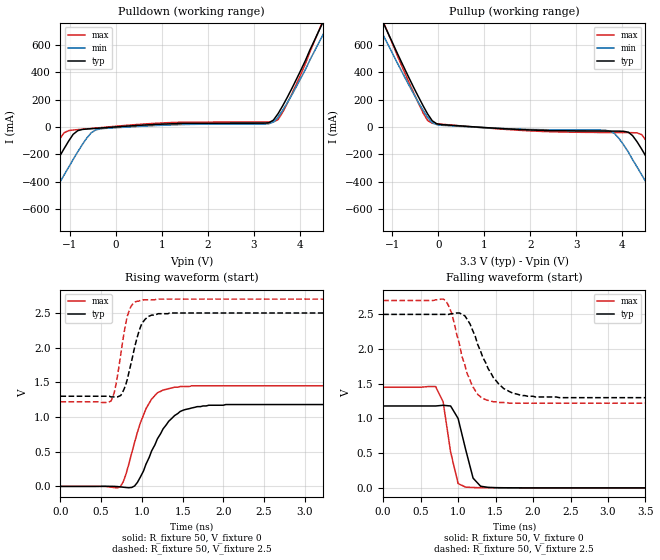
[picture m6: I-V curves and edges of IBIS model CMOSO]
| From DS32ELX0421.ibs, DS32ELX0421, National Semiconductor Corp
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|   Model CMOSO
[Model]  CMOSO
Model_type Output
Enable   Active-High
Vmeas =  1
C_comp   71.84fF   68.08fF   75.60fF
[Temperature Range]   25.0000   85.0000   -40.0000
[Voltage Range]   3.3000V   3.0000V   3.4650V
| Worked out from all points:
|   slope of the pulldown table from 0 to 0.495 V, typ, clamps not added: 44.3 ohm
|   slope of the pullup table from 0 to 0.495 V, typ, clamps not added: 36.2 ohm
|   rising waveform, R_fixture 50, V_fixture 0: 20-80 % time 310ps typ, NA min, 238ps max; typ from 0 V to 1.18 V
|   rising waveform, R_fixture 50, V_fixture 2.5: 20-80 % time 151ps typ, NA min, 123ps max; typ from 1.3 V to 2.5 V
|   falling waveform, R_fixture 50, V_fixture 0: 20-80 % time 164ps typ, NA min, 139ps max; typ from 1.18 V to 0 V
|   falling waveform, R_fixture 50, V_fixture 2.5: 20-80 % time 312ps typ, NA min, 231ps max; typ from 2.5 V to 1.3 V
[Pulldown]
|Voltage   I(typ)   I(min)   I(max)
-3.3V     -1.59A     -1.67A     -1.61A
-2.21V    -858mA     -1A        -788mA
-2.01V    -726mA     -883mA     -640mA
-1.72V    -530mA     -703mA     -424mA
-1.22V    -216mA     -408mA     -89.8mA
-1.02V    -102mA     -293mA     -26.7mA
-627mV    -15.2mA    -80.9mA    -14mA
-330mV    -8.06mA    -13.8mA    -5.07mA
3.43V     50.2mA     35.9mA     37.2mA
3.63V     154mA      121mA      107mA
4.52V     775mA      682mA      785mA
6.5V      2.23A      2.01A      2.41A
|6.60E+00   2.30E+00   2.08E+00   2.49E+00
[Pullup]
|Voltage   I(typ)   I(min)   I(max)
-3.2V     2.23A      2.01A      2.41A
-1.22V    775mA      682mA      785mA
-1.12V    703mA      617mA      705mA
-330mV    153mA      120mA      101mA
-132mV    44.3mA     30.8mA     26.6mA
3.73V     -30.5mA    -30.3mA    -40.8mA
4.13V     -38.6mA    -184mA     -41.7mA
4.42V     -163mA     -350mA     -56.7mA
5.02V     -530mA     -703mA     -426mA
5.31V     -726mA     -883mA     -640mA
5.41V     -792mA     -943mA     -714mA
6.6V      -1.59A     -1.67A     -1.61A
|-3.30E+00   2.30E+00   2.08E+00   2.49E+00
[Ramp]
|variable   typ   min   max
dV/dt_r   156.00m/266.4p   155.98m/289.5p   155.97m/245.7p
dV/dt_f   156.025m/256.2p  156.016m/278.8p   155.988m/237.1p
R_load  = 50
[Rising Waveform]
R_fixture=   50
V_fixture=   0
V_fixture_min=  0
V_fixture_max=  0
|time   V(typ)   V(min)   V(max)
0s        683pV      NA         627pV
735ps     -7.06mV    NA         -3.5mV
805ps     -16.2mV    NA         178mV
910ps     5.69mV     NA         634mV
1.05ns    320mV      NA         1.12V
1.19ns    685mV      NA         1.35V
1.4ns     1.02V      NA         1.43V
1.68ns    1.15V      NA         1.45V
2.03ns    1.18V      NA         1.45V
10ns      1.18V      NA         1.45V
[Rising Waveform]
R_fixture=   50
V_fixture=   2.5
V_fixture_min=  2.3
V_fixture_max=  2.7
|time   V(typ)   V(min)   V(max)
0s        1.3V       NA         1.22V
620ps     1.29V      NA         1.23V
680ps     1.29V      NA         1.46V
740ps     1.31V      NA         1.9V
820ps     1.54V      NA         2.45V
880ps     1.84V      NA         2.62V
960ps     2.22V      NA         2.67V
1.02ns    2.38V      NA         2.69V
1.34ns    2.5V       NA         2.7V
10ns      2.5V       NA         2.7V
[Falling Waveform]
R_fixture=   50
V_fixture=   0
V_fixture_min=  0
V_fixture_max=  0
|time   V(typ)   V(min)   V(max)
0s        1.18V      NA         1.45V
700ps     1.18V      NA         1.46V
800ps     1.19V      NA         1.24V
900ps     1.18V      NA         517mV
1ns       1V         NA         61.9mV
1.1ns     556mV      NA         11mV
1.2ns     140mV      NA         4.73mV
1.3ns     23.7mV     NA         3.08mV
1.4ns     6.86mV     NA         2.63mV
10ns      559nV      NA         420nV
[Falling Waveform]
R_fixture=   50
V_fixture=   2.5
V_fixture_min=  2.3
V_fixture_max=  2.7
|time   V(typ)   V(min)   V(max)
0s        2.5V       NA         2.7V
840ps     2.5V       NA         2.69V
910ps     2.51V      NA         2.53V
1.09ns    2.48V      NA         1.77V
1.19ns    2.28V      NA         1.47V
1.3ns     1.97V      NA         1.31V
1.47ns    1.59V      NA         1.24V
1.68ns    1.39V      NA         1.22V
2.03ns    1.31V      NA         1.22V
10ns      1.3V       NA         1.22V
